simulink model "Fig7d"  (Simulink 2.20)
settings: Solver=ode45  StartTime=0.0  StopTime=10.0  RelTol=1e-3  AbsTol=1e-6
libraries: simulink x1

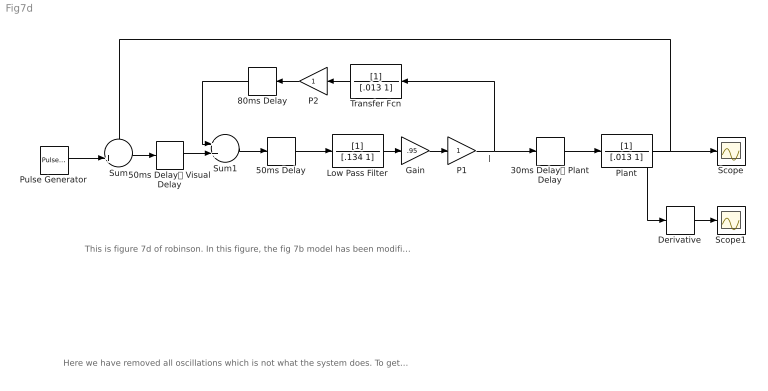
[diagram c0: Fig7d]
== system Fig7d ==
  note: 
  note: This is figure 7d of robinson. In this figure, the fig 7b model has been modified to remove the temporal mismath in 7b. This is accomplished by assing the 80msec delay to the inner feedback loop. P1 and P2 are variable gain elements to account for Lance O's adaptation data
  note: Here we have removed all oscillations which is not what the system does. To get good oscillations with this model (as in the real system) you need to either change the delay in the feedback loop or to adjust gains P1 and P2, Note that if you mess with P1 you have to mess with P2 to keep overall gain at 0.95 The problem is that you can only really get the model to ring at 2Hz which is way to low. The other failure is that oscillation ampl will depend on initial slip signal linearly, which it dont in the real world.
  30ms Delay Plant Delay : TransportDelay  DelayTime=.030  InitialInput=0  BufferSize=1024
  50ms Delay : TransportDelay  DelayTime=.050  InitialInput=0  BufferSize=1024
  50ms Delay Visual Delay : TransportDelay  DelayTime=.050  InitialInput=0  BufferSize=1024
  80ms Delay : TransportDelay  Orientation=left  DelayTime=.080  InitialInput=0  BufferSize=1024
  Derivative : Derivative
  Gain : Gain  Gain=.95
  Low Pass Filter : TransferFcn  Numerator=[1]  Denominator=[.134 1]
  P1 : Gain  Gain=1
  P2 : Gain  Orientation=left  Gain=1
  Plant : TransferFcn  Numerator=[1]  Denominator=[.013 1]
  Pulse Generator : simulink/Sources/Pulse Generator  period=100  duty=50  amplitude=20  start=0
  Scope : Scope
  Scope1 : Scope
  Sum : Sum  Inputs=-+
  Sum1 : Sum  Inputs=++
  Transfer Fcn : TransferFcn  Orientation=left  Numerator=[1]  Denominator=[.013 1]
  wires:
  Pulse Generator/1 -> Sum/2
  Low Pass Filter/1 -> Gain/1
  50ms Delay/1 -> Low Pass Filter/1
  Sum1/1 -> 50ms Delay/1
  Sum/1 -> 50ms Delay Visual Delay/1
  50ms Delay Visual Delay/1 -> Sum1/2
  80ms Delay/1 -> Sum1/1
  Transfer Fcn/1 -> P2/1
  P2/1 -> 80ms Delay/1
  Gain/1 -> P1/1
  Plant/1 -> Scope/1, Sum/1, Derivative/1
  30ms Delay Plant Delay/1 -> Plant/1
  Derivative/1 -> Scope1/1
  P1/1 -> 30ms Delay Plant Delay/1, Transfer Fcn/1
